(* Logix 5000 AddOnInstructionDefinition export AMCI_SD4840E2_Home_CCW; software revision 20.03 *)

ADD_ON_INSTRUCTION AMCI_SD4840E2_Home_CCW   (* revision 5.0, vendor AMCI, ExecuteEnableInFalse *)
// Revision note:
// Version 5.0 added the (hidden) ability to program the motor current and unlatched the error bit if the rung goes false.
VAR_INPUT
   Axis_Status_Bits : INT; {required}
   Type_0_for_standard_1_for_indexed : BOOL;
   Programmed_Speed : DINT; {required}
   Acceleration : INT; {required}
   Deceleration : INT; {required}
   motor_current : INT;
   Jerk : INT;
END_VAR
VAR_IN_OUT
   AMCI_SD4840E2_output_data : _000A:SD4840E2_4342D302:O:0; {required}
END_VAR
VAR_OUTPUT
   EN : BOOL; {access Read Only, visible}
   ER : BOOL; {access Read Only, visible}
END_VAR
VAR
   Upper_Result_X_1000 : DINT;
   command_data_block : INT[10];
        [0]   // Command Bits MSW
        [1]   // Command Bits LSW
        [2]   // Upper Target Position
        [3]   // Lower Target Position
        [4]   // Upper Programmed Speed
        [5]   // Lower Programmed Speed
END_VAR

ROUTINE EnableInFalse   (* ladder *)
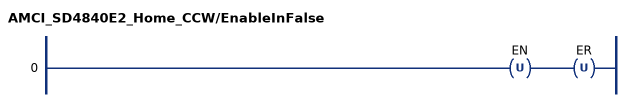
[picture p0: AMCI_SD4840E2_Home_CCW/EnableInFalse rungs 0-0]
   0: OTU(EN)OTU(ER);
END_ROUTINE

ROUTINE Logic   (* ladder *)
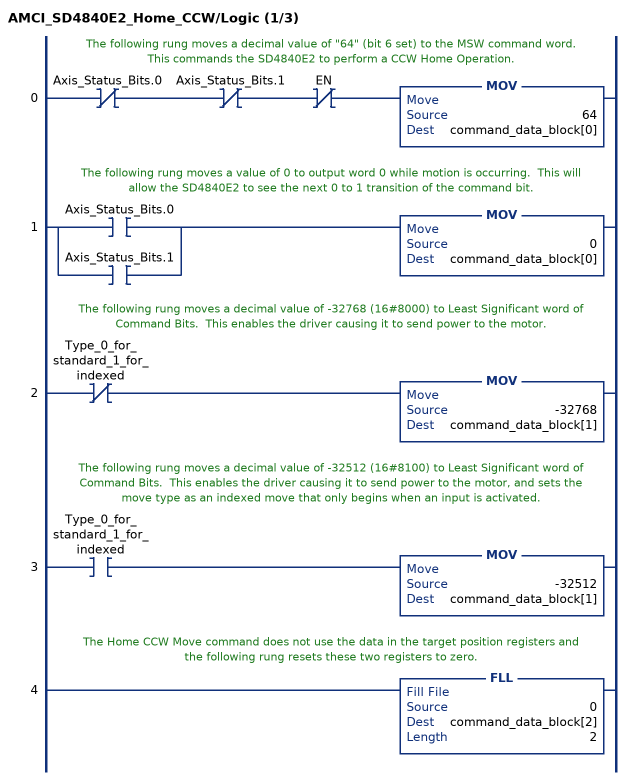
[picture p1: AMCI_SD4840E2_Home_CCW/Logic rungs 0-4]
   // The following rung moves a decimal value of "64" (bit 6 set) to the MSW command word.  This commands the SD4840E2 to perform a CCW Home Operation.
   0: XIO(Axis_Status_Bits.0)XIO(Axis_Status_Bits.1)XIO(EN)MOV(64,command_data_block[0]);
   // The following rung moves a value of 0 to output word 0 while motion is occurring.  This will allow the SD4840E2 to see the next 0 to 1 transition of the command bit.
   1: [XIC(Axis_Status_Bits.0) ,XIC(Axis_Status_Bits.1) ]MOV(0,command_data_block[0]);
   // The following rung moves a decimal value of -32768 (16#8000) to Least Significant word of Command Bits.  This enables the driver causing it to send power to the motor.
   2: XIO(Type_0_for_standard_1_for_indexed)MOV(-32768,command_data_block[1]);
   // The following rung moves a decimal value of -32512 (16#8100) to Least Significant word of Command Bits.  This enables the driver causing it to send power to the motor, and sets the move type as an indexed move that only begins when an input is activated.
   3: XIC(Type_0_for_standard_1_for_indexed)MOV(-32512,command_data_block[1]);
   // The Home CCW Move command does not use the data in the target position registers and the following rung resets these two registers to zero.
   4: FLL(0,command_data_block[2],2);
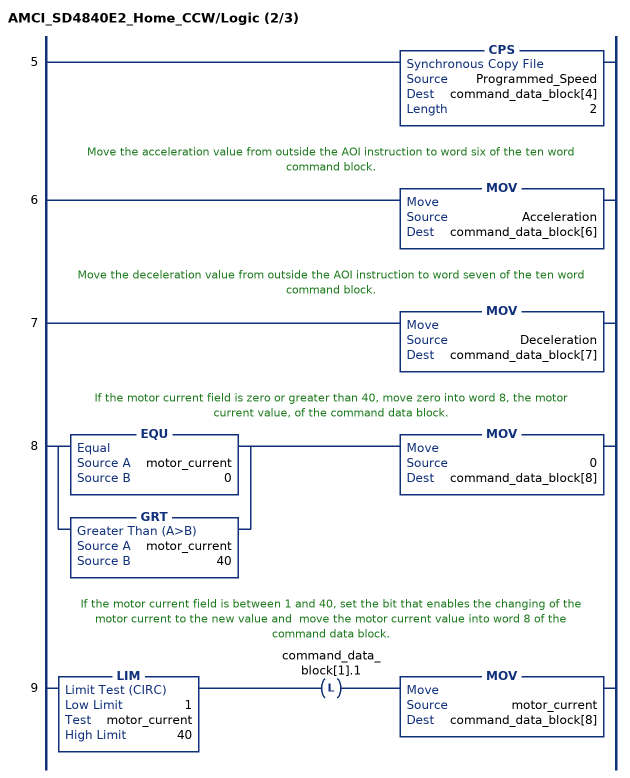
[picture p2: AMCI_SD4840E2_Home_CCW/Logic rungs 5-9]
   5: CPS(Programmed_Speed,command_data_block[4],2);
   // Move the acceleration value from outside the AOI instruction to word six of the ten word command block.
   6: MOV(Acceleration,command_data_block[6]);
   // Move the deceleration value from outside the AOI instruction to word seven of the ten word command block.
   7: MOV(Deceleration,command_data_block[7]);
   // If the motor current field is zero or greater than 40, move zero into word 8, the motor current value, of the command data block.
   8: [EQU(motor_current,0) ,GRT(motor_current,40) ]MOV(0,command_data_block[8]);
   // If the motor current field is between 1 and 40, set the bit that enables the changing of the motor current to the new value and  move the motor current value into word 8 of the command data block.
   9: LIM(1,motor_current,40)OTL(command_data_block[1].1)MOV(motor_current,command_data_block[8]);
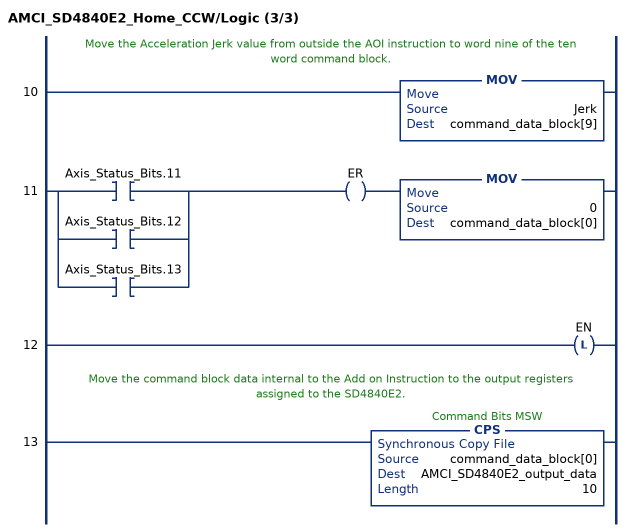
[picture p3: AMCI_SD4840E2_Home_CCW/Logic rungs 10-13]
   // Move the Acceleration Jerk value from outside the AOI instruction to word nine of the ten word command block.
   10: MOV(Jerk,command_data_block[9]);
   11: [XIC(Axis_Status_Bits.11) ,XIC(Axis_Status_Bits.12) ,XIC(Axis_Status_Bits.13) ]OTE(ER)MOV(0,command_data_block[0]);
   12: OTL(EN);
   // Move the command block data internal to the Add on Instruction to the output registers assigned to the SD4840E2.
   13: CPS(command_data_block[0],AMCI_SD4840E2_output_data,10);
END_ROUTINE
END_ADD_ON_INSTRUCTION
